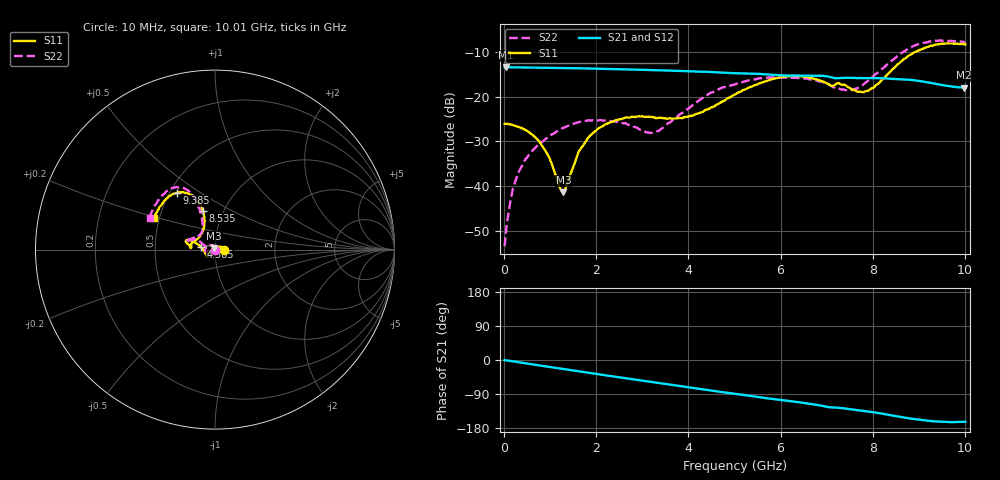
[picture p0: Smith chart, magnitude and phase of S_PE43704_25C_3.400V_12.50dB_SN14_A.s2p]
! Device ID: PE43704
! Dir: z:\PE43704\PE43704_Char_1_20130516\PE43704\AMB\3p400V\12p50dB
! Serial: 14
! Insertion: A
! Impedance: 50 ohm
! Temp: Amb
! VDD: 3.400V
! Attenuation Step: 12.50dB
! IDD: 1.139244e-01mA
#  Hz  S  RI  R  50
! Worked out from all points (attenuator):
!   401 points, 10 MHz to 10.01 GHz, reference 50 ohm
!   highest |S21| = -13.45 dB at 35 MHz (marker M1); lowest = -18.0 dB at 9.985 GHz (marker M2)
!   lowest |S11| = -41.4 dB at 1.285 GHz (marker M3), VSWR 1.02, Z = 49.5 + j0.709 ohm
!   |S11| at or under -10 dB: start of sweep to 8.936 GHz
!   |S22| runs from -53.4 to -7.5 dB; largest |S21 - S12| = 0.0016
!   S11 on the Smith chart (normalised r, x): 10 MHz: 1.10, +0.00; 4.585 GHz: 0.85, +0.02; 8.535 GHz: 0.80, +0.37; 9.385 GHz: 0.54, +0.40; 10.01 GHz: 0.47, +0.19
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1e7  0.0496 0.000183  0.2126 -0.000795  0.2127 -0.000739  0.00208 0.000434
3.5e7  0.0496 0.000958  0.2125 -0.00256  0.2125 -0.0027  0.00229 0.00168
1.85e8  0.0478 0.00581  0.2116 -0.0132  0.2115 -0.0132  0.00161 0.00894
4.1e8  0.042 0.012  0.2089 -0.0292  0.209 -0.0285  -0.00268 0.0175
8.35e8  0.0218 0.0169  0.2021 -0.0564  0.2021 -0.0563  -0.0185 0.0253
1.285e9  -0.00467 0.00716  0.1905 -0.0842  0.1906 -0.084  -0.0406 0.0188
1.685e9  -0.0253 -0.00937  0.1769 -0.1066  0.1769 -0.1065  -0.0528 0.00478
2.01e9  -0.0359 -0.0227  0.1638 -0.1231  0.1638 -0.123  -0.0537 -0.00581
2.385e9  -0.0408 -0.0343  0.1467 -0.14  0.1468 -0.1401  -0.0516 -0.0116
3.36e9  -0.046 -0.0353  0.0954 -0.1718  0.0955 -0.1716  -0.041 0.00626
3.91e9  -0.0568 -0.0153  0.0641 -0.1813  0.0643 -0.1812  -0.063 0.0265
4.585e9  -0.0782 0.0142  0.0252 -0.1848  0.0253 -0.1848  -0.1023 0.0557
5.01e9  -0.1002 0.0325  0.00247 -0.1822  0.00279 -0.1824  -0.1263 0.0544
5.96e9  -0.1532 0.0544  -0.0439 -0.1673  -0.0435 -0.1674  -0.1542 0.0519
6.685e9  -0.1572 0.035  -0.0764 -0.1528  -0.0763 -0.1528  -0.145 0.0528
7.56e9  -0.1075 0.0513  -0.1051 -0.1226  -0.1053 -0.1226  -0.0771 0.0909
7.885e9  -0.0766 0.0866  -0.1154 -0.1117  -0.1151 -0.1124  -0.0684 0.1311
8.36e9  -0.0592 0.1752  -0.1296 -0.0908  -0.1294 -0.0914  -0.0849 0.2222
8.535e9  -0.0689 0.2173  -0.1338 -0.0811  -0.1331 -0.0822  -0.103 0.2637
9.385e9  -0.2125 0.3169  -0.1314 -0.042  -0.1316 -0.0417  -0.252 0.3345
9.985e9  -0.3348 0.1844  -0.1199 -0.0364  -0.1209 -0.0365  -0.3596 0.1859
1.001e10  -0.3402 0.1743  -0.1203 -0.0369  -0.1211 -0.0373  -0.3637 0.1774
